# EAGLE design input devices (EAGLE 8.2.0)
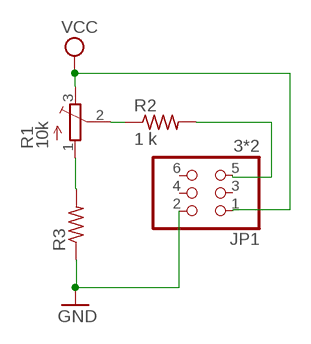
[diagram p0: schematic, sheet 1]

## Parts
JP1  3*2  PINHD-2X3-SMD  [2X03SMD]
R1  10k  TRIM_EU-SM-42/43A  [SM-42/43A]
R2  1 k  R-US_R1206  [R1206]
R3  R-US_R1206  [R1206]

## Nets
GND: JP1.2 R3.1
N$1: R1.2(S) R2.1
N$2: R1.1(A) R3.2
N$3: JP1.5 R2.2
VCC: JP1.1 R1.3(E)
Unconnected: JP1.3 JP1.4 JP1.6

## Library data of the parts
JP1 = fab:PINHD-2X3-SMD: PIN HEADER
R1 = pot:TRIM_EU-: POTENTIOMETER
R2 R3 = rcl:R-US_: RESISTOR, American symbol

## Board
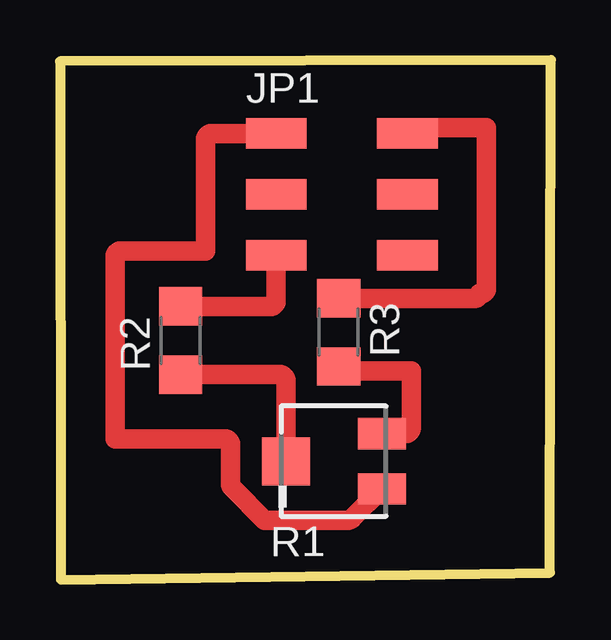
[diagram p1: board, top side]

Size 20.47 x 21.67 mm. Coordinates in mm from the lower left corner, seen from the top.
Outline: 0.04,0 20.43,0.29 20.47,21.67 0,21.61 0.04,0
Copper layers (1*16): Top 0.035mm / dielectric 1.5mm / Bottom 0.035mm
Design rules "default": minimum track width 10mil, minimum drill 24mil, track to track 8mil, track to pad 8mil, pad to pad 8mil, via to via 8mil, smd to smd 8mil, copper to edge 40mil, drill to drill 8mil, minimum pad ring 10mil, minimum via ring 8mil, stop-mask expansion 4mil, vias tented up to drill 0mil, thermal gap 10mil

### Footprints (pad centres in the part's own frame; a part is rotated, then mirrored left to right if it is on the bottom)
2X03SMD = smd 2.54 x 1.27: 1 -2.54,2.54; 2 2.92,2.54; 3 -2.54,0; 4 2.92,0; 5 -2.54,-2.54; 6 2.92,-2.54
SM-42/43A = smd 2 x 1.3: 1 2,1.15; 3 2,-1.15 | smd 2 x 2: 2 -2,0
R1206 = smd 1.6 x 1.803: 1 -1.422,0; 2 1.422,0

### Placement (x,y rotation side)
JP1  11.56,16.06 0 top
R1  11.42,4.94 0 top
R2  5.03,9.97 90 top
R3  11.62,10.31 270 top

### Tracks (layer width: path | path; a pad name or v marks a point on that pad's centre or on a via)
GND
  Top 0.813: R3.1 17.29,11.73 arc90 17.48,11.92 17.54,11.92 arc90 17.79,12.17 17.79,18.84 14.72,18.84 arc90 JP1.2
N$1
  Top 0.813: R2.1 9.17,8.55 arc-90 9.42,8.29 R1.2
N$2
  Top 0.813: R1.1 14.4,6.09 arc90 14.65,6.34 14.65,8.71 11.8,8.71 arc-90 R3.2
N$3
  Top 0.813: R2.2 8.77,11.39 arc90 9.02,11.65 JP1.5
VCC
  Top 0.813: JP1.1 6.32,18.6 arc90 6.07,18.35 6.07,13.71 2.55,13.71 arc90 2.3,13.46 2.3,5.87 6.87,5.87 arc-90 7.12,5.62 7.12,4 arc45 7.19,3.83 8.54,2.48 12.01,2.48 arc45 12.18,2.55 R1.3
